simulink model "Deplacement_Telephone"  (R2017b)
settings: Solver=ode15s  StartTime=0.0  StopTime=5  MaxStep=0.05  RelTol=1e-3  EnableMultiTasking=on
undefined symbols (not defined in the file): magnitude
libraries: simulink x1

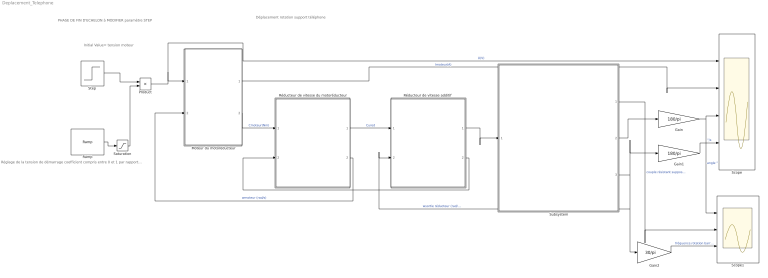
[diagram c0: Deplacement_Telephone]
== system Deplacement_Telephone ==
  note: Réglage de la tension de démarrage coefficient compris entre 0 et 1 par rapport à ' initial input ex 0.25*(6V de l'autre bloc)= tension de démarrage à 1.5V
  note: Initial Value= tension moteur
  note: Déplacement rotation support téléphone
  note: PHASE DE FIN D'ECHELON à MODIFIER paramètre STEP
  Gain : Gain  Gain=180/pi
  Gain1 : Gain  Gain=180/pi
  Gain2 : Gain  Gain=30/pi
  Moteur du motoréducteur : Subsystem  mask{R=0.5, K=0}
      mask prompts: R "Résistance interne"; K "K  en Nm/A ou V/(rad/s)"
  Product : Product
  Ramp : simulink/Sources/Ramp  slope=1.5  start=0  X0=1
  "Réducteur de vitesse additif " : Subsystem  mask{KR=1/1, rend=1}
      mask prompts: KR "Rapport de réduction ws/we"; rend "rendement du réducteur"
  Réducteur de vitesse du motoréducteur : Subsystem  mask{KR=1/1, rend=1}
      mask prompts: KR "Rapport de réduction ws/we"; rend "rendement du réducteur"
  Saturation : Saturate  UpperLimit=1  LowerLimit=0
  Scope : Scope  NumInputPorts=4
  Scope1 : Scope  NumInputPorts=3
  Step : Step  Time=3  Before=6  After=0  SampleTime=0
  Subsystem : Subsystem  mask{m=1, long=1, larg=1}
      mask prompts: m "masse en Kg portable+ support"; long "longueur  du support"; larg "Largueur du support"
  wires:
  Moteur du motoréducteur/2(cumot) -> Réducteur de vitesse du motoréducteur/1(Cmot)  "Cmoteur(Nm)"
  Réducteur de vitesse du motoréducteur/2(Wmoteur) -> Moteur du motoréducteur/2(rad/s)  "wmoteur (rad/s)"
  Product/1 -> Scope/1, Moteur du motoréducteur/1(U(v))  "U(V)"
  Gain/1 -> Scope1/1, Scope/3  "angle °"
  Step/1 -> Product/1
  Ramp/1 -> Saturation/1
  Moteur du motoréducteur/1(I(A)) -> Scope/2  "Imoteur(A)"
  Gain1/1 -> Scope/4  "°/s"
  Subsystem/3(vitesse angulaire sortie bras rad/s) -> Gain1/1, "Réducteur de vitesse additif "/2(W sort), Gain2/1  "wsortie réducteur (rad/s)"
  Réducteur de vitesse du motoréducteur/1(Csortie) -> "Réducteur de vitesse additif "/1(Cmot)  "Cured"
  Subsystem/2(Angle rad) -> Gain/1
  Gain2/1 -> Scope1/3  "fréquence rotation barre  trs/min"
  "Réducteur de vitesse additif "/2(Wmoteur) -> Réducteur de vitesse du motoréducteur/2(W sort)
  "Réducteur de vitesse additif "/1(Csortie) -> Subsystem/1(Cured)
  Subsystem/1(Couple Nm) -> Scope1/2  "couple résistant supposé  en Nmt"
  Saturation/1 -> Product/2

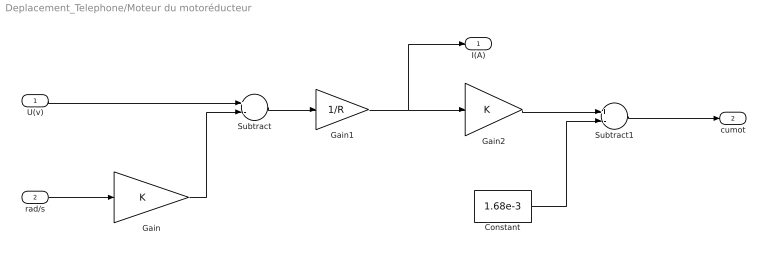
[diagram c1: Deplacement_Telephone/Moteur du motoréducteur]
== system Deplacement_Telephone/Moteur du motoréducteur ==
  U(v) : Inport
  rad/s : Inport  Port=2
  Constant : Constant  Value=1.68e-3
  Gain : Gain  Gain=K
  Gain1 : Gain  Gain=1/R
  Gain2 : Gain  Gain=K
  Subtract : Sum  Inputs=+-
  Subtract1 : Sum  Inputs=+-
  I(A) : Outport
  cumot : Outport  Port=2
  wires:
  U(v)/1 -> Subtract/1
  rad/s/1 -> Gain/1
  Gain/1 -> Subtract/2
  Subtract/1 -> Gain1/1
  Gain1/1 -> I(A)/1, Gain2/1
  Gain2/1 -> Subtract1/1
  Constant/1 -> Subtract1/2
  Subtract1/1 -> cumot/1

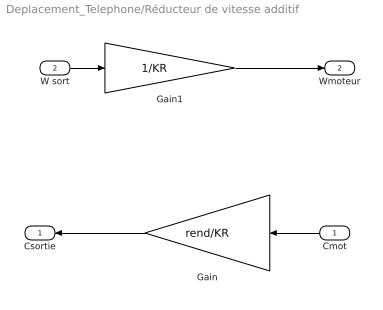
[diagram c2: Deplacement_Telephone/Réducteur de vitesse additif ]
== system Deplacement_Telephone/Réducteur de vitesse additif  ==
  Cmot : Inport
  W sort : Inport  Port=2
  Gain : Gain  Gain=rend/KR
  Gain1 : Gain  Gain=1/KR
  Csortie : Outport
  Wmoteur : Outport  Port=2
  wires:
  Cmot/1 -> Gain/1
  Gain/1 -> Csortie/1
  W sort/1 -> Gain1/1
  Gain1/1 -> Wmoteur/1

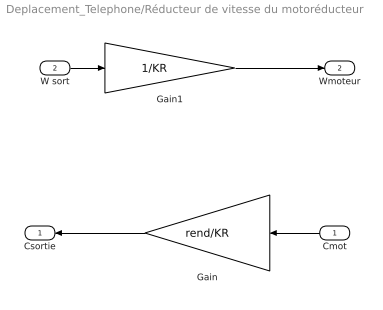
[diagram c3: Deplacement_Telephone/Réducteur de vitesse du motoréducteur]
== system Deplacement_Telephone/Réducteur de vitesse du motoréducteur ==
  Cmot : Inport
  W sort : Inport  Port=2
  Gain : Gain  Gain=rend/KR
  Gain1 : Gain  Gain=1/KR
  Csortie : Outport
  Wmoteur : Outport  Port=2
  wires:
  Cmot/1 -> Gain/1
  Gain/1 -> Csortie/1
  W sort/1 -> Gain1/1
  Gain1/1 -> Wmoteur/1

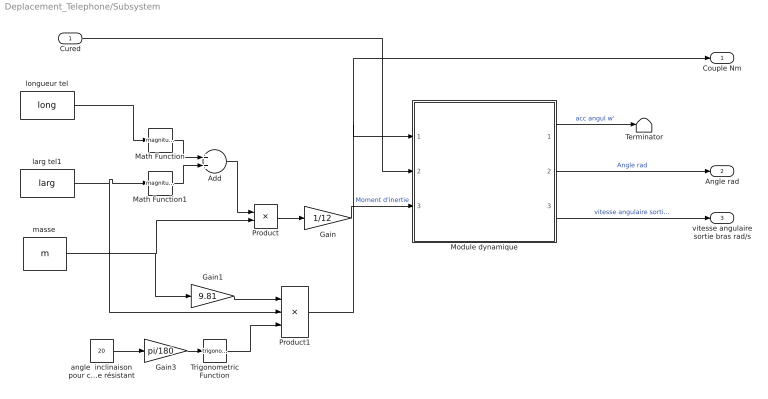
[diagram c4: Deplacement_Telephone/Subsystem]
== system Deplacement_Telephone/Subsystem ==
  Cured : Inport
  Add : Sum
  Gain : Gain  Gain=1/12
  Gain1 : Gain  Gain=9.81
  Gain3 : Gain  Gain=pi/180
  Math Function : Math  Operator=magnitude^2
  Math Function1 : Math  Operator=magnitude^2
  Module dynamique : Subsystem
  Product : Product
  Product1 : Product  Inputs=3
  Terminator : Terminator
  Trigonometric Function : Trigonometry
  angle  inclinaison pour calculer un couple résistant : Constant  Value=20
  larg tel1 : Constant  Value=larg
  longueur tel : Constant  Value=long
  "masse " : Constant  Value=m
  Couple Nm : Outport
  Angle rad : Outport  Port=2
  vitesse angulaire sortie bras rad/s : Outport  Port=3
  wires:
  Module dynamique/2(teta rad) -> Angle rad/1  "Angle rad"
  Gain/1 -> Module dynamique/3(J)  "Moment d'inertie"
  Cured/1 -> Module dynamique/2(Cured)
  Module dynamique/3(W (rad/s)) -> vitesse angulaire sortie bras rad/s/1  "vitesse angulaire sortie bras rad/s"
  "masse "/1 -> Gain1/1, Product/2
  Module dynamique/1(acc) -> Terminator/1  "acc angul w'"
  longueur tel/1 -> Math Function/1
  larg tel1/1 -> Product1/2, Math Function1/1
  Math Function/1 -> Add/1
  Math Function1/1 -> Add/2
  Add/1 -> Product/1
  Product/1 -> Gain/1
  Gain1/1 -> Product1/1
  angle  inclinaison pour calculer un couple résistant/1 -> Gain3/1
  Gain3/1 -> Trigonometric Function/1
  Trigonometric Function/1 -> Product1/3
  Product1/1 -> Couple Nm/1, Module dynamique/1(Cr)

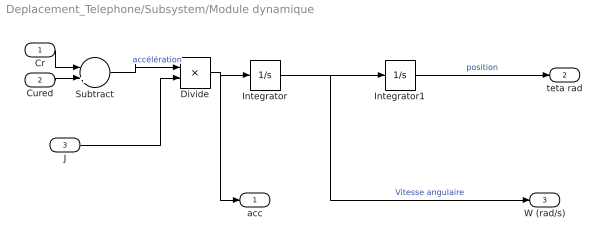
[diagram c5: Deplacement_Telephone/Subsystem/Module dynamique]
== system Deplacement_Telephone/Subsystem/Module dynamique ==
  Cr : Inport
  Cured : Inport  Port=2
  J : Inport  Port=3
  Divide : Product  Inputs=*/
  Integrator : Integrator
  Integrator1 : Integrator
  Subtract : Sum  Inputs=-+
  acc : Outport
  teta rad : Outport  Port=2
  W (rad/s) : Outport  Port=3
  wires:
  Integrator/1 -> Integrator1/1, W (rad/s)/1  "Vitesse angulaire"
  Cr/1 -> Subtract/1
  Integrator1/1 -> teta rad/1  "position"
  Cured/1 -> Subtract/2
  Subtract/1 -> Divide/1  "accélération"
  Divide/1 -> Integrator/1, acc/1
  J/1 -> Divide/2
